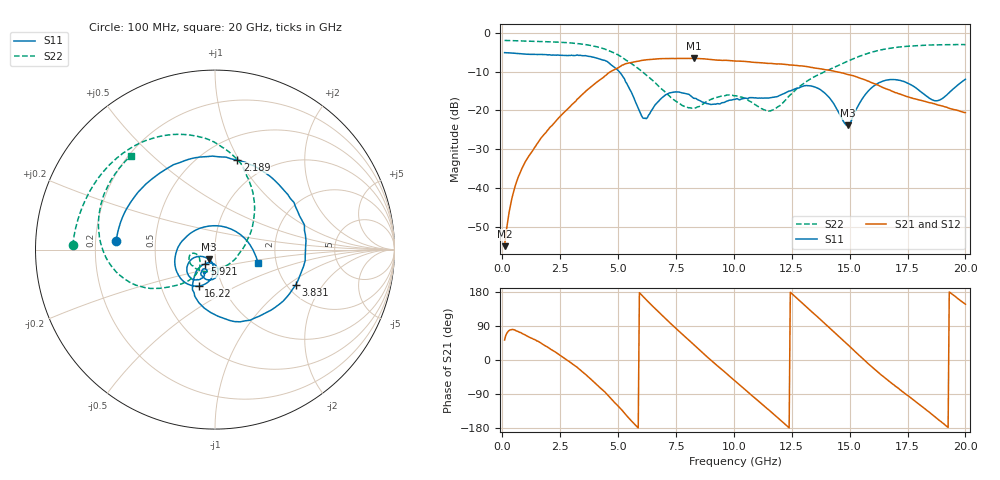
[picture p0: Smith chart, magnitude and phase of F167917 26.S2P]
!  2-Port S-parameters saved by WinCal
! VAR MeasName=S-Parameters (CALIBRATED_DATA) read from VNA (N5242A)
! VAR MeasDate=2016-11-22 9:01:00
! VAR NAME=F167917 26
! VAR FILENAME=F167917 26.S2P
! VAR DATE=2016-11-22 9:01:00
! VAR PHYS_PORTS=1,2
# Hz S DB R 50
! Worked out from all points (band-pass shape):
!   401 points, 100 MHz to 20 GHz, reference 50 ohm
!   highest |S21| = -6.60 dB at 8.259 GHz (marker M1); lowest = -54.9 dB at 100 MHz (marker M2)
!   |S21| within 3 dB of the highest: 4.81 GHz to 14.06 GHz (9.253 GHz wide, 98.1 % of centre)
!   lowest |S11| = -23.9 dB at 14.93 GHz (marker M3), VSWR 1.14, Z = 46.4 - j5.06 ohm
!   |S11| at or under -10 dB: 5.044 GHz to end of sweep
!   |S22| runs from -20.2 to -2.0 dB; largest |S21 - S12| = 0.0047
!   S11 on the Smith chart (normalised r, x): 100 MHz: 0.29, +0.04; 2.189 GHz: 0.72, +0.98; 3.831 GHz: 2.21, -1.16; 5.921 GHz: 0.88, -0.14; 16.22 GHz: 0.77, -0.33; 20 GHz: 1.60, -0.26
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1e8  -5.16 175.3  -54.86 52.7  -54.84 51.1  -2.03 178.3
7.4675e8  -5.42 145.5  -36.34 73.0  -36.25 72.8  -2.13 168.1
2.1895e9  -5.76 76.0  -23.58 25.2  -23.58 25.0  -2.40 144.8
3.43325e9  -5.92 2.4  -16.02 -29.8  -16.02 -29.7  -2.95 119.6
3.83125e9  -6.19 -23.9  -13.91 -50.9  -13.90 -50.8  -3.33 109.8
4.478e9  -7.31 -67.0  -10.96 -87.4  -10.92 -87.4  -4.35 91.8
4.9755e9  -9.58 -100.3  -9.14 -119.8  -9.09 -120.0  -5.65 76.9
5.92075e9  -20.11 -125.8  -7.29 177.6  -7.27 177.5  -9.45 49.2
6.21925e9  -22.13 -97.9  -6.99 158.9  -6.98 158.7  -10.92 40.1
6.7665e9  -17.54 -83.5  -6.72 125.8  -6.72 125.8  -13.86 21.1
8.259e9  -16.85 -121.1  -6.60 41.1  -6.58 41.2  -19.37 -75.0
9.055e9  -18.43 -115.8  -6.94 -3.0  -6.92 -3.0  -17.08 -121.8
1.005e10  -17.16 -112.5  -7.30 -55.2  -7.29 -55.1  -16.25 -158.5
1.09455e10  -16.76 -116.5  -7.68 -102.3  -7.63 -102.3  -18.61 -169.8
1.199025e10  -16.11 -112.2  -8.06 -157.2  -8.01 -157.2  -18.76 -135.9
1.338325e10  -13.81 -137.2  -8.96 126.3  -8.94 126.5  -11.66 -133.8
1.49255e10  -23.85 -122.2  -10.77 40.2  -10.72 40.4  -7.33 -150.0
1.6219e10  -13.05 -114.1  -13.45 -31.4  -13.43 -31.0  -4.63 -171.3
1.67165e10  -12.10 -134.0  -14.72 -56.6  -14.68 -56.3  -4.05 179.7
1.77115e10  -13.62 178.1  -16.86 -103.1  -16.74 -103.2  -3.42 163.2
1.875625e10  -17.52 86.5  -18.47 -153.7  -18.41 -153.2  -3.15 147.9
2e10  -11.99 -17.6  -20.55 147.2  -20.40 147.7  -3.09 131.8
